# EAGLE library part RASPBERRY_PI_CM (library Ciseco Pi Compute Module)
Raspberry Pi Compute Module As anounced in this blog post http://www.raspberrypi.org/raspberry-pi-compute-module-new-product/ Based on infomation from this schematic http://www.raspberrypi.org/wp-content/uploads/2014/04/RPI-CM-V1_1-SCHEMATIC.pdf Footprint is unproven and no matching part confimed as of yet
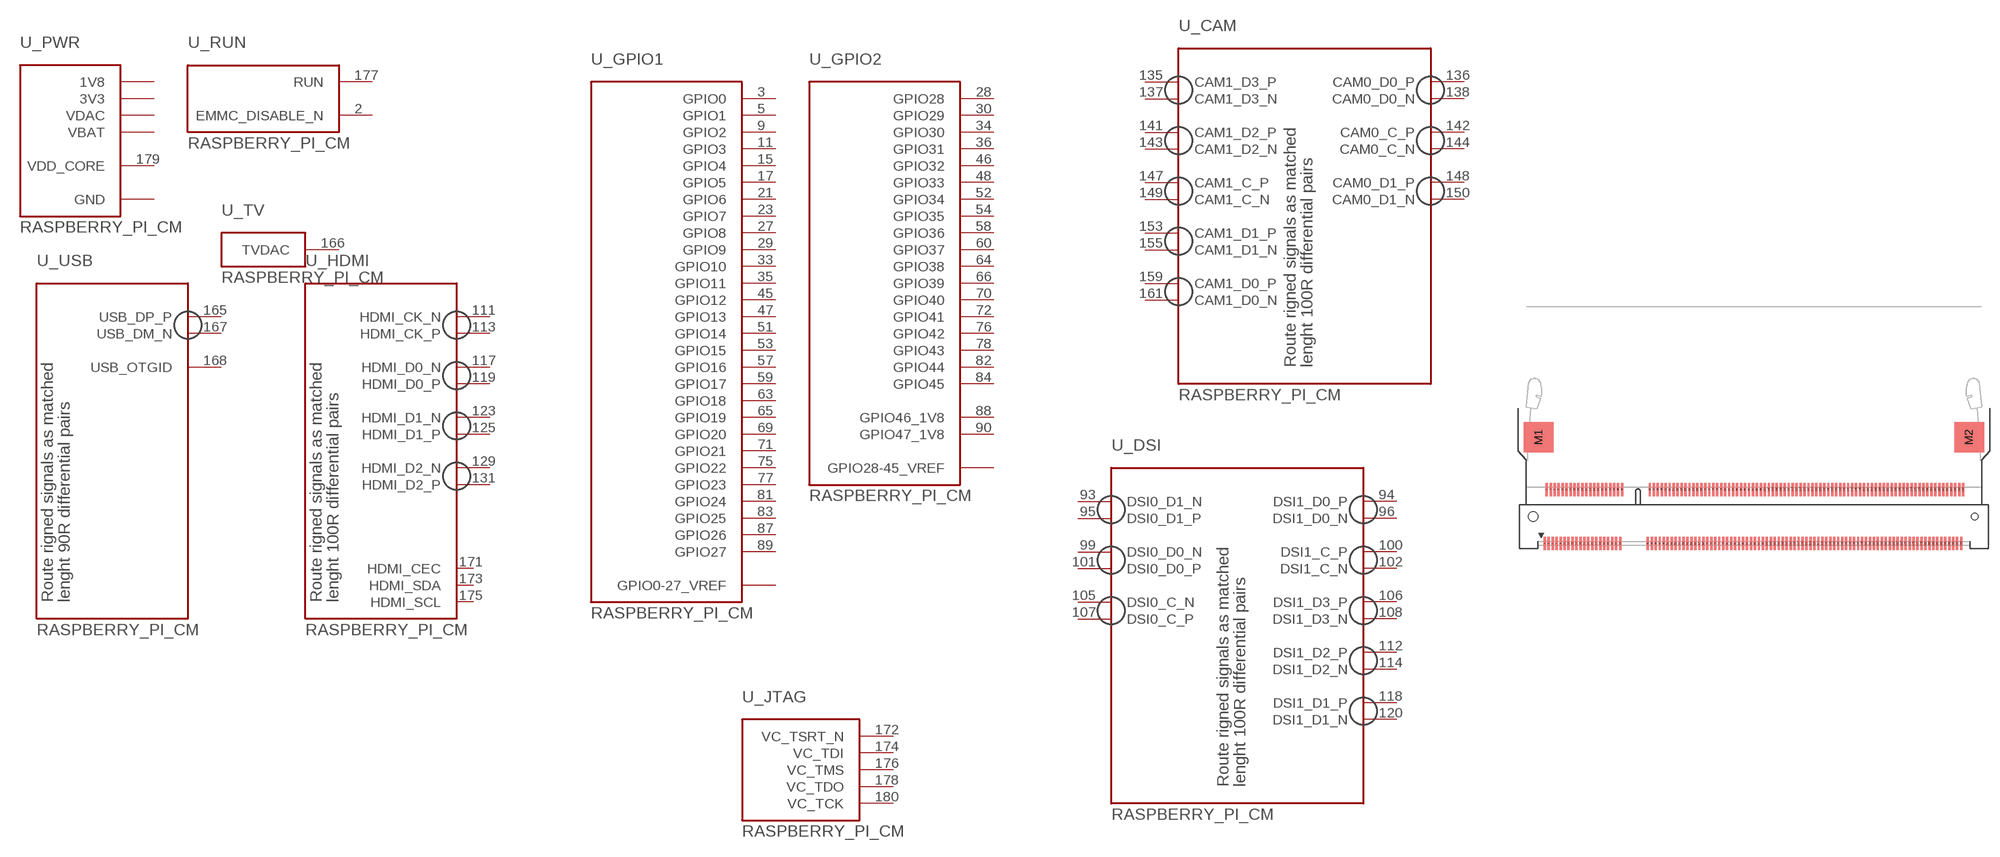
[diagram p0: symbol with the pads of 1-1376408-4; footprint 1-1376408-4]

Designator prefix U; gates _PWR=CM_PWR _RUN=CM_RUN _USB=CM_USB _TV=CM_TV _HDMI=CM_HDMI _GPIO1=CM_GPIO1 _GPIO2=CM_GPIO2 _CAM=CM_CAM _DSI=CM_DSI _JTAG=CM_JTAG

## RASPBERRY_PI_CM-1-1376408-4  [1-1376408-4]
1  _PWR:GND
2  _RUN:EMMC_DISABLE_N
3  _GPIO1:GPIO0
5  _GPIO1:GPIO1
7  _PWR:GND
9  _GPIO1:GPIO2
11  _GPIO1:GPIO3
13  _PWR:GND
15  _GPIO1:GPIO4
17  _GPIO1:GPIO5
19  _PWR:GND
21  _GPIO1:GPIO6
23  _GPIO1:GPIO7
25  _PWR:GND
26  _PWR:GND
27  _GPIO1:GPIO8
28  _GPIO2:GPIO28
29  _GPIO1:GPIO9
30  _GPIO2:GPIO29
31  _PWR:GND
32  _PWR:GND
33  _GPIO1:GPIO10
34  _GPIO2:GPIO30
35  _GPIO1:GPIO11
36  _GPIO2:GPIO31
37  _PWR:GND
38  _PWR:GND
39  _GPIO1:GPIO0-27_VREF
40  _GPIO1:GPIO0-27_VREF
41  _GPIO2:GPIO28-45_VREF
42  _GPIO2:GPIO28-45_VREF
43  _PWR:GND
44  _PWR:GND
45  _GPIO1:GPIO12
46  _GPIO2:GPIO32
47  _GPIO1:GPIO13
48  _GPIO2:GPIO33
49  _PWR:GND
50  _PWR:GND
51  _GPIO1:GPIO14
52  _GPIO2:GPIO34
53  _GPIO1:GPIO15
54  _GPIO2:GPIO35
55  _PWR:GND
56  _PWR:GND
57  _GPIO1:GPIO16
58  _GPIO2:GPIO36
59  _GPIO1:GPIO17
60  _GPIO2:GPIO37
61  _PWR:GND
62  _PWR:GND
63  _GPIO1:GPIO18
64  _GPIO2:GPIO38
65  _GPIO1:GPIO19
66  _GPIO2:GPIO39
67  _PWR:GND
68  _PWR:GND
69  _GPIO1:GPIO20
70  _GPIO2:GPIO40
71  _GPIO1:GPIO21
72  _GPIO2:GPIO41
73  _PWR:GND
74  _PWR:GND
75  _GPIO1:GPIO22
76  _GPIO2:GPIO42
77  _GPIO1:GPIO23
78  _GPIO2:GPIO43
79  _PWR:GND
80  _PWR:GND
81  _GPIO1:GPIO24
82  _GPIO2:GPIO44
83  _GPIO1:GPIO25
84  _GPIO2:GPIO45
85  _PWR:GND
86  _PWR:GND
87  _GPIO1:GPIO26
88  _GPIO2:GPIO46_1V8
89  _GPIO1:GPIO27
90  _GPIO2:GPIO47_1V8
91  _PWR:GND
92  _PWR:GND
93  _DSI:DSI0_D1_N
94  _DSI:DSI1_D0_P
95  _DSI:DSI0_D1_P
96  _DSI:DSI1_D0_N
97  _PWR:GND
98  _PWR:GND
99  _DSI:DSI0_D0_N
100  _DSI:DSI1_C_P
101  _DSI:DSI0_D0_P
102  _DSI:DSI1_C_N
103  _PWR:GND
104  _PWR:GND
105  _DSI:DSI0_C_N
106  _DSI:DSI1_D3_P
107  _DSI:DSI0_C_P
108  _DSI:DSI1_D3_N
109  _PWR:GND
110  _PWR:GND
111  _HDMI:HDMI_CK_N
112  _DSI:DSI1_D2_P
113  _HDMI:HDMI_CK_P
114  _DSI:DSI1_D2_N
115  _PWR:GND
116  _PWR:GND
117  _HDMI:HDMI_D0_N
118  _DSI:DSI1_D1_P
119  _HDMI:HDMI_D0_P
120  _DSI:DSI1_D1_N
121  _PWR:GND
122  _PWR:GND
123  _HDMI:HDMI_D1_N
125  _HDMI:HDMI_D1_P
127  _PWR:GND
129  _HDMI:HDMI_D2_N
131  _HDMI:HDMI_D2_P
133  _PWR:GND
134  _PWR:GND
135  _CAM:CAM1_D3_P
136  _CAM:CAM0_D0_P
137  _CAM:CAM1_D3_N
138  _CAM:CAM0_D0_N
139  _PWR:GND
140  _PWR:GND
141  _CAM:CAM1_D2_P
142  _CAM:CAM0_C_P
143  _CAM:CAM1_D2_N
144  _CAM:CAM0_C_N
145  _PWR:GND
146  _PWR:GND
147  _CAM:CAM1_C_P
148  _CAM:CAM0_D1_P
149  _CAM:CAM1_C_N
150  _CAM:CAM0_D1_N
151  _PWR:GND
152  _PWR:GND
153  _CAM:CAM1_D1_P
155  _CAM:CAM1_D1_N
157  _PWR:GND
159  _CAM:CAM1_D0_P
161  _CAM:CAM1_D0_N
163  _PWR:GND
164  _PWR:GND
165  _USB:USB_DP_P
166  _TV:TVDAC
167  _USB:USB_DM_N
168  _USB:USB_OTGID
169  _PWR:GND
170  _PWR:GND
171  _HDMI:HDMI_CEC
172  _JTAG:VC_TSRT_N
173  _HDMI:HDMI_SDA
174  _JTAG:VC_TDI
175  _HDMI:HDMI_SCL
176  _JTAG:VC_TMS
177  _RUN:RUN
178  _JTAG:VC_TDO
179  _PWR:VDD_CORE
180  _JTAG:VC_TCK
181  _PWR:GND
182  _PWR:GND
183  _PWR:1V8
184  _PWR:1V8
185  _PWR:1V8
186  _PWR:1V8
187  _PWR:GND
188  _PWR:GND
189  _PWR:VDAC
190  _PWR:VDAC
191  _PWR:3V3
192  _PWR:3V3
193  _PWR:3V3
194  _PWR:3V3
195  _PWR:GND
196  _PWR:GND
197  _PWR:VBAT
198  _PWR:VBAT
199  _PWR:VBAT
200  _PWR:VBAT

## Footprint 1-1376408-4 (pad centres in mm)
DDR2 SODIMM SOCKET 0.6mm Pitch 200 Pos. Connector for Kontron X-Board 2.5V Source: http://catalog.tycoelectronics.com ... JPN_CD_1376408_S.pdf
smd 0.35 x 2: 1 -32.65,-4.1; 2 -32.35,4.1; 3 -32.05,-4.1; 4 -31.75,4.1; 5 -31.45,-4.1; 6 -31.15,4.1; 7 -30.85,-4.1; 8 -30.55,4.1; 9 -30.25,-4.1; 10 -29.95,4.1; 11 -29.65,-4.1; 12 -29.35,4.1; 13 -29.05,-4.1; 14 -28.75,4.1; 15 -28.45,-4.1; 16 -28.15,4.1; 17 -27.85,-4.1; 18 -27.55,4.1; 19 -27.25,-4.1; 20 -26.95,4.1; 21 -26.65,-4.1; 22 -26.35,4.1; 23 -26.05,-4.1; 24 -25.75,4.1; 25 -25.45,-4.1; 26 -25.15,4.1; 27 -24.85,-4.1; 28 -24.55,4.1; 29 -24.25,-4.1; 30 -23.95,4.1; 31 -23.65,-4.1; 32 -23.35,4.1; 33 -23.05,-4.1; 34 -22.75,4.1; 35 -22.45,-4.1; 36 -22.15,4.1; 37 -21.85,-4.1; 38 -21.55,4.1; 39 -21.25,-4.1; 40 -20.95,4.1; 41 -17.05,-4.1; 42 -16.75,4.1; 43 -16.45,-4.1; 44 -16.15,4.1; 45 -15.85,-4.1; 46 -15.55,4.1; 47 -15.25,-4.1; 48 -14.95,4.1; 49 -14.65,-4.1; 50 -14.35,4.1; 51 -14.05,-4.1; 52 -13.75,4.1; 53 -13.45,-4.1; 54 -13.15,4.1; 55 -12.85,-4.1; 56 -12.55,4.1; 57 -12.25,-4.1; 58 -11.95,4.1; 59 -11.65,-4.1; 60 -11.35,4.1; 61 -11.05,-4.1; 62 -10.75,4.1; 63 -10.45,-4.1; 64 -10.15,4.1; 65 -9.85,-4.1; 66 -9.55,4.1; 67 -9.25,-4.1; 68 -8.95,4.1; 69 -8.65,-4.1; 70 -8.35,4.1; 71 -8.05,-4.1; 72 -7.75,4.1; 73 -7.45,-4.1; 74 -7.15,4.1; 75 -6.85,-4.1; 76 -6.55,4.1; 77 -6.25,-4.1; 78 -5.95,4.1; 79 -5.65,-4.1; 80 -5.35,4.1; 81 -5.05,-4.1; 82 -4.75,4.1; 83 -4.45,-4.1; 84 -4.15,4.1; 85 -3.85,-4.1; 86 -3.55,4.1; 87 -3.25,-4.1; 88 -2.95,4.1; 89 -2.65,-4.1; 90 -2.35,4.1; 91 -2.05,-4.1; 92 -1.75,4.1; 93 -1.45,-4.1; 94 -1.15,4.1; 95 -0.85,-4.1; 96 -0.55,4.1; 97 -0.25,-4.1; 98 0.05,4.1; 99 0.35,-4.1; 100 0.65,4.1; 101 0.95,-4.1; 102 1.25,4.1; 103 1.55,-4.1; 104 1.85,4.1; 105 2.15,-4.1; 106 2.45,4.1; 107 2.75,-4.1; 108 3.05,4.1; 109 3.35,-4.1; 110 3.65,4.1; 111 3.95,-4.1; 112 4.25,4.1; 113 4.55,-4.1; 114 4.85,4.1; 115 5.15,-4.1; 116 5.45,4.1; 117 5.75,-4.1; 118 6.05,4.1; 119 6.35,-4.1; 120 6.65,4.1; 121 6.95,-4.1; 122 7.25,4.1; 123 7.55,-4.1; 124 7.85,4.1; 125 8.15,-4.1; 126 8.45,4.1; 127 8.75,-4.1; 128 9.05,4.1; 129 9.35,-4.1; 130 9.65,4.1; 131 9.95,-4.1; 132 10.25,4.1; 133 10.55,-4.1; 134 10.85,4.1; 135 11.15,-4.1; 136 11.45,4.1; 137 11.75,-4.1; 138 12.05,4.1; 139 12.35,-4.1; 140 12.65,4.1; 141 12.95,-4.1; 142 13.25,4.1; 143 13.55,-4.1; 144 13.85,4.1; 145 14.15,-4.1; 146 14.45,4.1; 147 14.75,-4.1; 148 15.05,4.1; 149 15.35,-4.1; 150 15.65,4.1; 151 15.95,-4.1; 152 16.25,4.1; 153 16.55,-4.1; 154 16.85,4.1; 155 17.15,-4.1; 156 17.45,4.1; 157 17.75,-4.1; 158 18.05,4.1; 159 18.35,-4.1; 160 18.65,4.1; 161 18.95,-4.1; 162 19.25,4.1; 163 19.55,-4.1; 164 19.85,4.1; 165 20.15,-4.1; 166 20.45,4.1; 167 20.75,-4.1; 168 21.05,4.1; 169 21.35,-4.1; 170 21.65,4.1; 171 21.95,-4.1; 172 22.25,4.1; 173 22.55,-4.1; 174 22.85,4.1; 175 23.15,-4.1; 176 23.45,4.1; 177 23.75,-4.1; 178 24.05,4.1; 179 24.35,-4.1; 180 24.65,4.1; 181 24.95,-4.1; 182 25.25,4.1; 183 25.55,-4.1; 184 25.85,4.1; 185 26.15,-4.1; 186 26.45,4.1; 187 26.75,-4.1; 188 27.05,4.1; 189 27.35,-4.1; 190 27.65,4.1; 191 27.95,-4.1; 192 28.25,4.1; 193 28.55,-4.1; 194 28.85,4.1; 195 29.15,-4.1; 196 29.45,4.1; 197 29.75,-4.1; 198 30.05,4.1; 199 30.35,-4.1; 200 30.65,4.1
smd 4.5 x 4.6: M1 -33.55,12; M2 31.55,12
hole 1.45 at -34.4,0
hole 0.95 at 32.4,0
